VAR_GLOBAL CONSTANT
	
	// input definition
	cChannels		: UDINT 	:= 3;    // number of input channels
	cOversamples 	: UDINT 	:= 10;	 // oversamples from input terminal
	
	// pupulation for statistical calculations
	cPupulation 	: UDINT     := 6000;	
	
	// Source MultiArray
	cBufferLength : UDINT := 100; 
	
	// wait for cAppendData MultiArrays with cBufferLength Elements before calculating | Elements in total = cPupulation 
	cAppendData     : UDINT := cPupulation/cBufferLength;

	
	// histogram
	cMaxBins		: UDINT 	:= 200;  // number of bins
	cLowerBinLimit	: LREAL 	:= -12;  // min limit of hist
	cUpperBinLimit  : LREAL     := 12;   // max limit of hist

	
	
	
END_VAR
